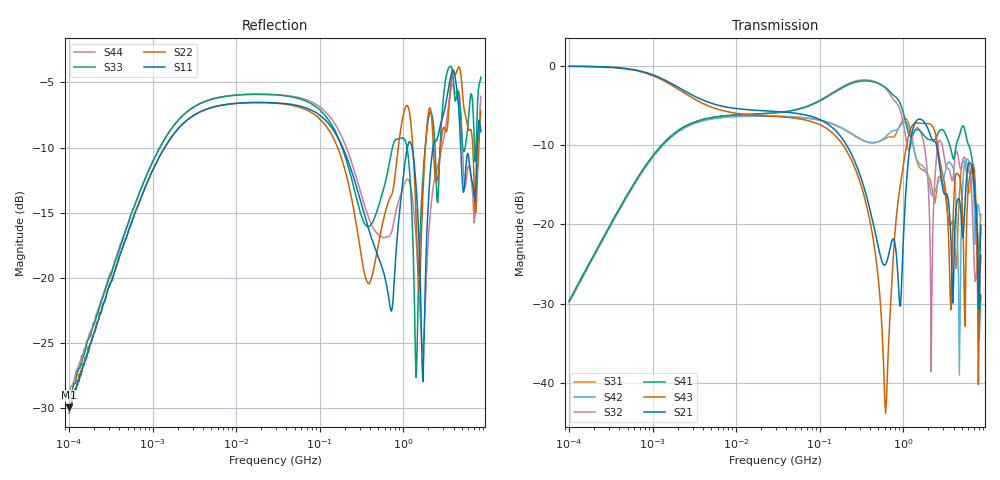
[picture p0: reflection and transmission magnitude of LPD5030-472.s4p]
# MHz S MA R 50
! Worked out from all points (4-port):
!   498 points, 100 kHz to 8.5 GHz, reference 50 ohm
!   strongest paths, dB at 100 kHz, 1.698 MHz, 29.49 MHz, 500.7 MHz, 8.5 GHz:
!     S21: -0.1, -2.3, -5.8, -22.7, -20.1
!     S43: -0.1, -2.5, -6.4, -26.6, -23.9
!     S41: -29.6, -8.8, -5.9, -2.2, -28.9
!     S32: -29.7, -8.8, -5.9, -2.2, -21.1
!     S42: -29.8, -8.9, -6.4, -9.6, -19.5
!     S31: -29.8, -8.9, -6.4, -9.6, -18.7
!   lowest |S11| = -29.9 dB at 100 kHz (marker M1), VSWR 1.07, Z = 50.3 + j3.19 ohm
!   |S11| at or under -10 dB: 188.7 MHz to 1.121 GHz (932.8 MHz wide, 142 % of centre); 1.275 GHz to 2.27 GHz (995 MHz wide, 56.1 % of centre); 4.879 GHz to 7.676 GHz (2.797 GHz wide, 44.6 % of centre)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
0.1  0.03195 83.3  0.9914 -1.9  0.03243 -94.5  0.03312 85.6
     0.9914 -1.9  0.03027 83.9  0.0329 86.0  0.03236 -94.8
     0.03243 -94.5  0.0329 86.0  0.03366 79.2  0.9899 -2.1
     0.03312 85.6  0.03236 -94.8  0.9899 -2.1  0.03613 83.8
3.775873  0.4349 20.7  0.6144 -17.2  0.4461 -159.9  0.4541 22.3
          0.6144 -17.2  0.4345 20.7  0.4546 22.4  0.4454 -160.0
          0.4461 -159.9  0.4546 22.4  0.4679 20.6  0.5862 -19.1
          0.4541 22.3  0.4454 -160.0  0.5862 -19.1  0.4684 20.5
355.4419  0.1683 -93.3  0.1572 -114.1  0.332 41.1  0.8019 -53.1
          0.1572 -114.1  0.09921 -65.8  0.8133 -58.0  0.3344 37.7
          0.332 41.1  0.8133 -58.0  0.1593 -59.6  0.1385 -126.8
          0.8019 -53.1  0.3344 37.7  0.1385 -126.8  0.1836 -91.9
614.9063  0.09794 -109.7  0.05611 -98.7  0.3487 -19.1  0.7269 -104.2
          0.05611 -98.7  0.1806 -50.6  0.7199 -114.2  0.3568 -20.2
          0.3487 -19.1  0.7199 -114.2  0.2354 -62.4  0.006472 106.8
          0.7269 -104.2  0.3568 -20.2  0.006472 106.8  0.143 -107.7
1306.515  0.3025 136.7  0.4007 -97.1  0.3264 173.5  0.3739 165.5
          0.4007 -97.1  0.3122 147.9  0.3615 158.6  0.3152 176.8
          0.3264 173.5  0.3615 158.6  0.1362 124.2  0.4243 -120.4
          0.3739 165.5  0.3152 176.8  0.4243 -120.4  0.1945 101.5
5383.342  0.2201 -2.7  0.1113 75.0  0.249 42.7  0.4052 -17.6
          0.1113 75.0  0.4389 -2.5  0.2653 -8.1  0.2369 52.3
          0.249 42.7  0.2653 -8.1  0.3057 44.0  0.03299 -66.9
          0.4052 -17.6  0.2369 52.3  0.03299 -66.9  0.2308 35.7
8500  0.3639 -39.8  0.09868 33.0  0.1167 14.0  0.03603 -2.2
      0.09868 33.0  0.4389 -34.2  0.08834 82.3  0.106 -23.9
      0.1167 14.0  0.08834 82.3  0.5884 -43.0  0.06379 48.2
      0.03603 -2.2  0.106 -23.9  0.06379 48.2  0.4969 -42.6
